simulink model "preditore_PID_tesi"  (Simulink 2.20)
settings: Solver=VariableStepDiscrete  StartTime=0.0  StopTime=16  RelTol=1e-3  AbsTol=1e-6
libraries: simulink x3, Puma x1

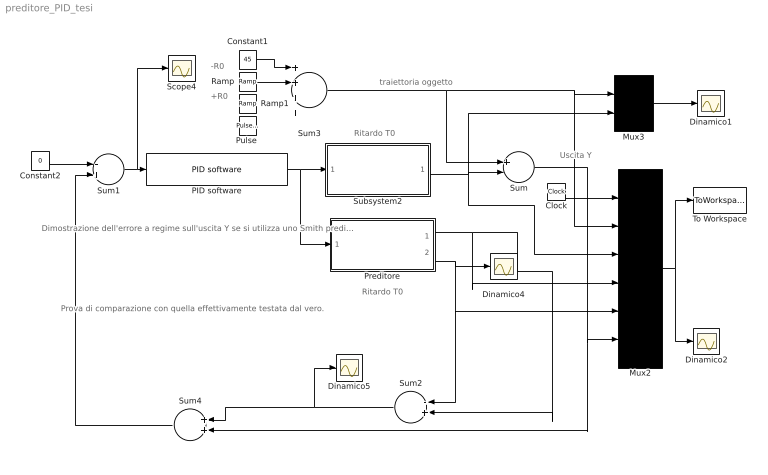
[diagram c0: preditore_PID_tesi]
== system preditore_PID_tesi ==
  note: traiettoria oggetto
  note: Dimostrazione dell'errore a regime sull'uscita Y se si utilizza uno Smith predictor nell'inseguire un oggetto in movimento. L'errore a regime DY=T0*R0 dove T0 = Ritardo sistema. R0= Ampiezza Rampa.
  note: -R0
  note: +R0
  note: Ritardo T0
  note: Ritardo T0
  note: Uscita Y
  note: Prova di comparazione con quella effettivamente testata dal vero.
  Clock : Clock
  Constant1 : Constant  Value=45
  Constant2 : Constant  Value=0
  Dinamico{1..2,4..5} (4 alike) : Scope
  Mux2 : Mux  Inputs=6
  Mux3 : Mux  Inputs=2
  PID software : Puma/PID software  Ti=1  Td=0.1  T=.130  Kp=0.5  N=10
  Preditore : Subsystem  mask(Modello del Puma 260 in Alter Mode){Ts=.260}
      mask prompts: Ts "Tempo di Campionamento Ts della seriale"
      mask help: Questo blocco racchiude il comportamento dinamico del Puma 260 pilotato dalla seriale. La rappresentazione e' a variabili di stato.
      mask init:
      | K=10; % attenuazione del guadagno puma.
      | A=[0,0,0,0,0,0,0,0,0,0;
      | 1,0,0,0,0,0,0,0,0,0;
      | 0,1,0,0,0,0,0,0,0,0;
      | 0,0,1,0,0,0,0,0,0,0;
      | 0,0,0,1,0,0,0,0,0,0;
      | 0,0,0,0,1,0,0,0,0,0;
      | 0,0,0,0,0,1,0,0,0,0;
      | 0,0,0,0,0,0,1,0,0,0;
      | 0,0,0,0,0,0,0,1,0,0;
      | 0,0,0,0,0,0,0,0,1/K,1];
      | B=[1;0;0;0;0;0;0;0;0;0];
      | C=[0,0,0,0,0,0,0,0,0,1;
      | 1/K,1/K,1/K,1/K,1/K,1/K,1/K,1/K,1/K,1];
      | D=[0;0];
  "Pulse " : simulink/Sources/Pulse Generator  period=30  duty=10  amplitude=-50  start=30
  Ramp : simulink/Sources/Ramp  slope=-26  start=7  X0=0
  Ramp1 : simulink/Sources/Ramp  slope=+26  start=25  X0=0
  Scope4 : Scope
  Subsystem2 : Subsystem  mask(Modello del Puma 260 in Alter Mode){Ts=.260}
      mask prompts: Ts "Tempo di Campionamento Ts della seriale"
      mask help: Questo blocco racchiude il comportamento dinamico del Puma 260 pilotato dalla seriale. La rappresentazione e' a variabili di stato.
      mask init:
      | K=10; % attenuazione del guadagno puma.
      | A=[0,0,0,0,0,0,0,0,0,0;
      | 1,0,0,0,0,0,0,0,0,0;
      | 0,1,0,0,0,0,0,0,0,0;
      | 0,0,1,0,0,0,0,0,0,0;
      | 0,0,0,1,0,0,0,0,0,0;
      | 0,0,0,0,1,0,0,0,0,0;
      | 0,0,0,0,0,1,0,0,0,0;
      | 0,0,0,0,0,0,1,0,0,0;
      | 0,0,0,0,0,0,0,1,0,0;
      | 0,0,0,0,0,0,0,0,1/K,1];
      | B=[1;0;0;0;0;0;0;0;0;0];
      | C=[0,0,0,0,0,0,0,0,0,1];
      | D=[0];
  Sum : Sum  Inputs=+-
  Sum1 : Sum  Inputs=-+
  Sum2 : Sum  Orientation=left  Inputs=-+
  Sum3 : Sum  Inputs=++++
  Sum4 : Sum  Orientation=left  Inputs=++
  To Workspace : ToWorkspace  VariableName=out  SampleTime=-1
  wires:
  Subsystem2/1(Out1) -> Sum/2, Mux3/2, Mux2/3
  Constant1/1 -> Sum3/1
  Preditore/2(Out2) -> Dinamico4/1, Sum2/1, Mux2/5
  Sum3/1 -> Sum/1, Mux3/1, Mux2/2
  Sum1/1 -> Scope4/1, PID software/1
  Sum4/1 -> Sum1/2
  Constant2/1 -> Sum1/1
  Sum2/1 -> Sum4/1, Dinamico5/1
  PID software/1 -> Subsystem2/1(In1), Preditore/1(In1)
  Ramp/1 -> Sum3/2
  Mux2/1 -> Dinamico2/1, To Workspace/1
  Mux3/1 -> Dinamico1/1
  Clock/1 -> Mux2/1
  Preditore/1(Out1) -> Sum2/2, Mux2/4
  Sum/1 -> Sum4/2, Mux2/6

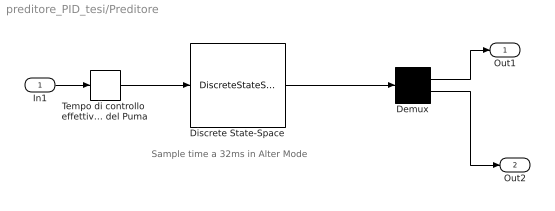
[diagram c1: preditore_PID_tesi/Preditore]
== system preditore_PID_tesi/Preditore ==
  note: Sample time a 32ms in Alter Mode
  In1 : Inport  Port=1  PortWidth=-1  SampleTime=-1
  Demux : Demux  Outputs=2
  Discrete State-Space : DiscreteStateSpace  A=A  B=B  C=C  D=D  X0=0  SampleTime=.033
  Tempo di controllo  effettivo Ts del Puma : ZeroOrderHold  SampleTime=Ts
  Out1 : Outport  Port=1
  Out2 : Outport  Port=2
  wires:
  In1/1 -> Tempo di controllo  effettivo Ts del Puma/1
  Discrete State-Space/1 -> Demux/1
  Tempo di controllo  effettivo Ts del Puma/1 -> Discrete State-Space/1
  Demux/1 -> Out1/1
  Demux/2 -> Out2/1

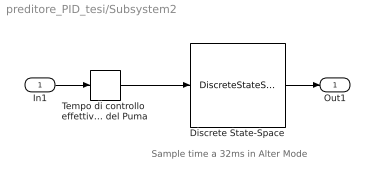
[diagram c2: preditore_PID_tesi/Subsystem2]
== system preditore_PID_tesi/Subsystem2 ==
  note: Sample time a 32ms in Alter Mode
  In1 : Inport  Port=1  PortWidth=-1  SampleTime=-1
  Discrete State-Space : DiscreteStateSpace  A=A  B=B  C=C  D=D  X0=0  SampleTime=.033
  Tempo di controllo  effettivo Ts del Puma : ZeroOrderHold  SampleTime=Ts
  Out1 : Outport  Port=1
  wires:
  In1/1 -> Tempo di controllo  effettivo Ts del Puma/1
  Discrete State-Space/1 -> Out1/1
  Tempo di controllo  effettivo Ts del Puma/1 -> Discrete State-Space/1
